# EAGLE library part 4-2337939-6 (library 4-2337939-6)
PCIE GEN4 CON,SMT,64POS,15u",MYLAR,ST Source: Datasheet
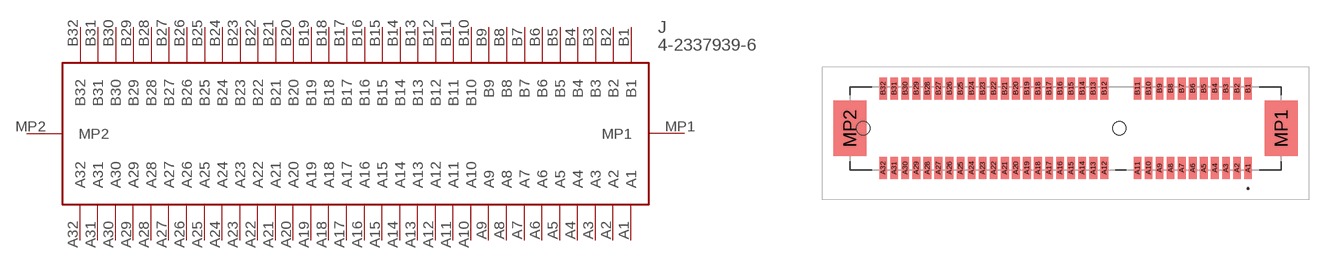
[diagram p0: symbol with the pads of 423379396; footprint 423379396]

Designator prefix J

## 4-2337939-6 (Description: PCIE GEN4 CON,SMT,64POS,15u",MYLAR,ST; Height: 11.25mm; Manufacturer_Name: TE Connectivity; Manufacturer_Part_Number: 4-2337939-6)  [423379396]
A1  A1
A2  A2
A3  A3
A4  A4
A5  A5
A6  A6
A7  A7
A8  A8
A9  A9
A10  A10
A11  A11
A12  A12
A13  A13
A14  A14
A15  A15
A16  A16
A17  A17
A18  A18
A19  A19
A20  A20
A21  A21
A22  A22
A23  A23
A24  A24
A25  A25
A26  A26
A27  A27
A28  A28
A29  A29
A30  A30
A31  A31
A32  A32
B1  B1
B2  B2
B3  B3
B4  B4
B5  B5
B6  B6
B7  B7
B8  B8
B9  B9
B10  B10
B11  B11
B12  B12
B13  B13
B14  B14
B15  B15
B16  B16
B17  B17
B18  B18
B19  B19
B20  B20
B21  B21
B22  B22
B23  B23
B24  B24
B25  B25
B26  B26
B27  B27
B28  B28
B29  B29
B30  B30
B31  B31
B32  B32
MP1  MP1
MP2  MP2

## Footprint 423379396 (pad centres in mm)
4-2337939-6-1
smd 0.7 x 2: A1 16.5,-3.6; A2 15.5,-3.6; A3 14.5,-3.6; A4 13.5,-3.6; A5 12.5,-3.6; A6 11.5,-3.6; A7 10.5,-3.6; A8 9.5,-3.6; A9 8.5,-3.6; A10 7.5,-3.6; A11 6.5,-3.6; A12 3.5,-3.6; A13 2.5,-3.6; A14 1.5,-3.6; A15 0.5,-3.6; A16 -0.5,-3.6; A17 -1.5,-3.6; A18 -2.5,-3.6; A19 -3.5,-3.6; A20 -4.5,-3.6; A21 -5.5,-3.6; A22 -6.5,-3.6; A23 -7.5,-3.6; A24 -8.5,-3.6; A25 -9.5,-3.6; A26 -10.5,-3.6; A27 -11.5,-3.6; A28 -12.5,-3.6; A29 -13.5,-3.6; A30 -14.5,-3.6; A31 -15.5,-3.6; A32 -16.5,-3.6; B1 16.5,3.6; B2 15.5,3.6; B3 14.5,3.6; B4 13.5,3.6; B5 12.5,3.6; B6 11.5,3.6; B7 10.5,3.6; B8 9.5,3.6; B9 8.5,3.6; B10 7.5,3.6; B11 6.5,3.6; B12 3.5,3.6; B13 2.5,3.6; B14 1.5,3.6; B15 0.5,3.6; B16 -0.5,3.6; B17 -1.5,3.6; B18 -2.5,3.6; B19 -3.5,3.6; B20 -4.5,3.6; B21 -5.5,3.6; B22 -6.5,3.6; B23 -7.5,3.6; B24 -8.5,3.6; B25 -9.5,3.6; B26 -10.5,3.6; B27 -11.5,3.6; B28 -12.5,3.6; B29 -13.5,3.6; B30 -14.5,3.6; B31 -15.5,3.6; B32 -16.5,3.6
smd 3 x 5: MP1 19.5,0; MP2 -19.5,0
hole 1.2 at 4.85,0
hole 1.2 at -18.3,0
